TYPE E_AnalysisIDs :
(
	(* analysis chain *)
	eID_Source := 1,
	eID_Histogram,
	eID_Mean,
	eID_Std,
	eID_Skew,
	eID_ExcessKurtosis,
	eID_Sink_Hist,
	eID_Sink_Mean,
	eID_Sink_Std,
	eID_Sink_Skew,
	eID_Sink_ExcessKurtosis
	
) UDINT;
END_TYPE
